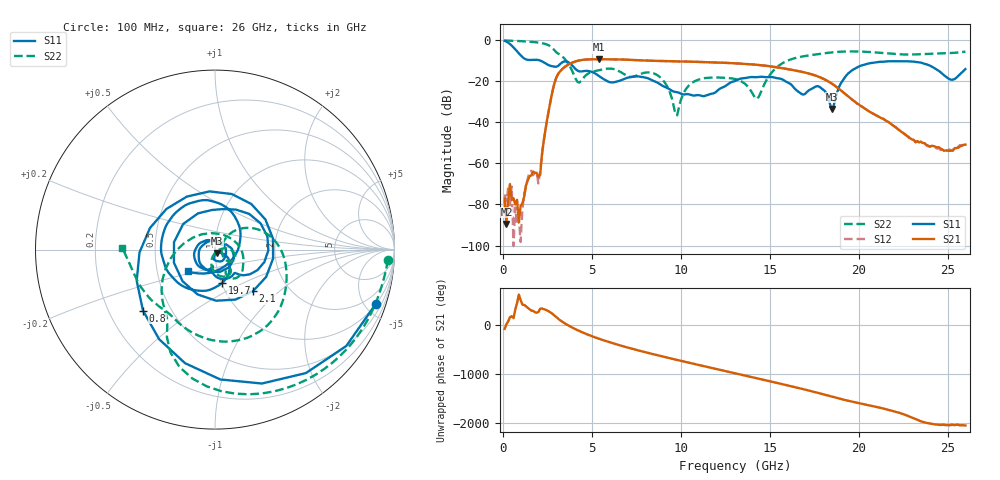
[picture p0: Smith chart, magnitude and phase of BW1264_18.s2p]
!Keysight Technologies,N5245B,MY57181159,A.13.60.06
!Date: Friday, December 18, 2020 23:52:51
!Correction: S11(Full 2 Port(1,2))
!S21(Full 2 Port(1,2))
!S12(Full 2 Port(1,2))
!S22(Full 2 Port(1,2))
!S2P File: Measurements: S11, S21, S12, S22:
# Hz S  dB  R 50
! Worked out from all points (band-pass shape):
!   260 points, 100 MHz to 26 GHz, reference 50 ohm
!   highest |S21| = -9.43 dB at 5.4 GHz (marker M1); lowest = -89.5 dB at 200 MHz (marker M2)
!   |S21| within 3 dB of the highest: 3.608 GHz to 14.62 GHz (11.02 GHz wide, 121 % of centre)
!   lowest |S11| = -33.6 dB at 18.5 GHz (marker M3), VSWR 1.04, Z = 50.8 - j1.93 ohm
!   |S11| at or under -10 dB: 2.072 GHz to end of sweep
!   |S22| runs from -36.6 to -0.3 dB; largest |S21 - S12| = 0.00053
!   S11 on the Smith chart (normalised r, x): 100 MHz: 1.04, -5.95; 800 MHz: 0.35, -0.33; 2.1 GHz: 1.33, -0.69; 19.7 GHz: 1.01, -0.39; 26 GHz: 0.72, -0.18
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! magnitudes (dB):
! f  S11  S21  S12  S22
! 100 MHz  -0.5  -77.1  -75.1  -0.3
! 200 MHz  -0.8  -89.5  -78.5  -0.4
! 300 MHz  -1.4  -78.1  -71.7  -0.4
! 400 MHz  -2.0  -70.1  -80.4  -0.4
! 500 MHz  -2.8  -77.9  -71.4  -0.5
! 800 MHz  -5.6  -77.8  -89.8  -0.6
! 1.5 GHz  -9.8  -66.4  -64.3  -0.9
! 2.1 GHz  -10.1  -65.6  -63.6  -1.5
! 3 GHz  -13.1  -18.5  -18.5  -6.0
! 4.5 GHz  -15.3  -9.7  -9.7  -18.9
! 5.4 GHz  -17.6  -9.4  -9.4  -14.8
! 8.8 GHz  -21.4  -10.3  -10.3  -17.9
! 9.8 GHz  -25.5  -10.4  -10.4  -36.6
! 10.7 GHz  -27.1  -10.7  -10.7  -20.6
! 13.1 GHz  -19.9  -11.4  -11.4  -19.2
! 14.3 GHz  -18.1  -12.2  -12.1  -28.6
! 15.5 GHz  -18.7  -13.5  -13.5  -12.7
! 17.4 GHz  -23.7  -16.9  -16.9  -7.3
! 18.5 GHz  -33.6  -21.3  -21.3  -6.1
! 19.7 GHz  -14.4  -29.5  -29.5  -5.6
! 21.7 GHz  -10.4  -40.1  -40.2  -6.6
! 26 GHz  -14.2  -51.0  -51.1  -5.7
